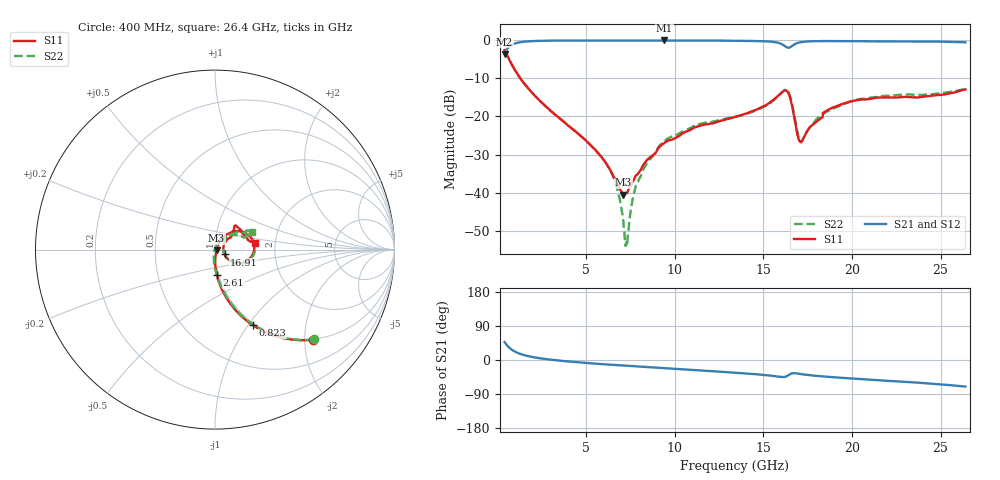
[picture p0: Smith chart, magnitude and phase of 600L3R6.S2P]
!  American Technical Ceramics  Date:  10/23/2012
!  One Norden Lane
!  Huntington Station,  NY.  11746-2102
!  Tel:  (631) 622-4700  Fax:  (631) 622-4748
!  Part Number  600L3R6	Mounting Orientation:  Vertical
!  Description:  Ultra Low ESR Microwave capacitors
!  Application:  Coupling, Bypass, Tuning, DC Block
!  Filters, Matching
# GHZ S DB R 50
! Freq  |S11|  S11 Ph  |S21|  S21 Ph  |S12|  S12 Ph  |S22|  S22 Ph
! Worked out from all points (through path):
!   801 points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, 400 MHz to 26.4 GHz, reference 50 ohm
!   highest |S21| = -0.04 dB at 9.403 GHz (marker M1); lowest = -3.6 dB at 400 MHz (marker M2)
!   group delay of S21, straight-line fit = 8.51 ps
!   lowest |S11| = -40.6 dB at 7.095 GHz (marker M3), VSWR 1.02, Z = 50.9 - j0.37 ohm
!   |S11| at or under -10 dB: 1.29 GHz to end of sweep
!   |S22| runs from -54.1 to -2.6 dB; largest |S21 - S12| = 0.0043
!   S11 on the Smith chart (normalised r, x): 400 MHz: 0.98, -2.20; 823 MHz: 0.97, -1.06; 2.61 GHz: 0.98, -0.29; 16.91 GHz: 1.11, -0.06; 26.4 GHz: 1.57, +0.12
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0.4  -2.58 -42.5  -3.56 47.3  -3.55 47.3  -2.56 -42.2
0.823  -6.52 -63.3  -1.13 26.6  -1.12 26.6  -6.50 -62.7
1.44  -10.96 -76.2  -0.39 13.7  -0.38 13.7  -10.93 -75.4
2.61  -16.88 -85.8  -0.12 3.2  -0.12 3.1  -16.87 -85.6
4.755  -25.35 -88.7  -0.04 -7.0  -0.04 -6.9  -25.40 -97.2
6.413  -34.47 -71.6  -0.06 -12.5  -0.04 -12.5  -34.69 -108.7
6.803  -38.01 -52.7  -0.07 -13.7  -0.04 -13.8  -39.94 -115.4
7.095  -40.56 -22.8  -0.07 -14.6  -0.05 -14.7  -47.25 -135.4
7.29  -40.16 1.5  -0.06 -15.1  -0.05 -15.3  -54.08 142.9
7.615  -37.17 27.7  -0.06 -16.1  -0.04 -16.3  -42.01 82.3
7.843  -35.36 36.9  -0.05 -16.8  -0.04 -17.0  -37.92 72.4
9.078  -28.30 62.5  -0.05 -20.4  -0.07 -20.6  -28.12 69.4
9.403  -27.01 60.6  -0.04 -21.5  -0.06 -21.6  -26.55 64.6
13.4  -20.14 53.8  -0.12 -33.4  -0.11 -33.5  -20.10 47.5
16.26  -13.17 4.0  -1.66 -43.9  -1.67 -43.9  -13.00 4.5
16.553  -15.84 -27.8  -1.72 -36.2  -1.72 -36.2  -15.42 -27.0
16.91  -24.46 -26.7  -0.72 -35.7  -0.73 -35.7  -23.86 -29.1
17.17  -26.47 13.2  -0.45 -37.5  -0.46 -37.5  -26.64 12.3
17.755  -22.28 36.8  -0.25 -40.8  -0.26 -40.8  -22.14 44.0
19.315  -16.97 44.8  -0.21 -46.7  -0.22 -46.7  -17.23 35.9
22.078  -15.01 45.6  -0.30 -55.2  -0.30 -55.2  -14.52 23.1
26.4  -12.91 9.4  -0.53 -70.2  -0.53 -70.1  -12.78 25.0
